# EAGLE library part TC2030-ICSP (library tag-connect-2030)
TAG-CONNECT ICSP Connector Manufacturer: Tag-Connect Cable for easy In-Circuit Serial Programming. Designed for Microchip ICD2, suitable for many others. Two variants - one "with legs" (for hands-free fit on PCB) and another "without legs" for quick programming. PADDescription 1MCLR/Vpp 2Vdd 3GND 4PGD (ISPDAT) 5PGC (ISPCLK) 6nc (used for LVP) ©2009 ROFA.cz - modified and updated by Robert Darlington &#8249;rdarlington@gmail.com&#8250;
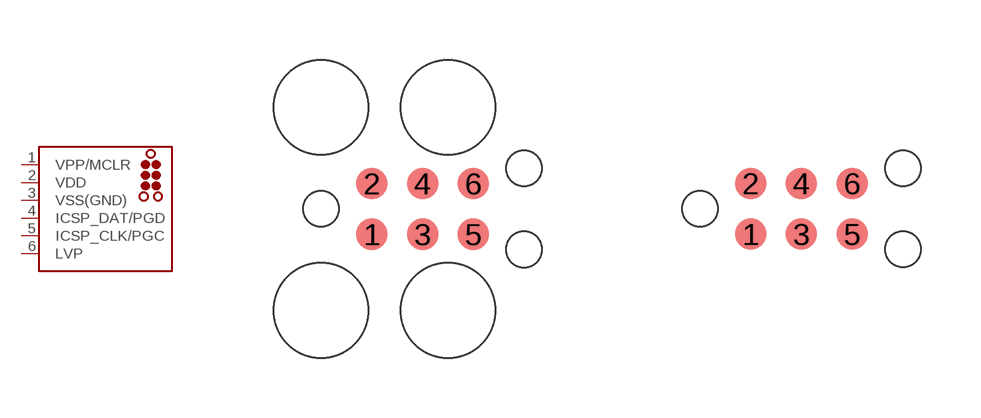
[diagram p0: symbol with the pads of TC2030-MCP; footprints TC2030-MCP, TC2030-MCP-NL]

Designator prefix J

## TC2030-ICSP-MCP  [TC2030-MCP]
1  VPP/MCLR  pas
2  VDD  pwr
3  VSS(GND)  pwr
4  ICSP_DAT/PGD
5  ICSP_CLK/PGC  out
6  LVP

## TC2030-ICSP-MCP-NL  [TC2030-MCP-NL]
Pads as for TC2030-MCP

## TC2030-ICSP  [TC2030-MCP-NL-CP]
Pads as for TC2030-MCP

## Footprint TC2030-MCP (pad centres in mm)
TAG-CONNECT ICSP Connector - Legged version Manufacturer: Tag-Connect Cable for easy In-Circuit Serial Programming. Designed for Microchip ICD2, suitable for many others. NOTE: Eagle's default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
smd 0.787 x 0.787: 1 1.27,-0.635; 2 1.27,0.635; 3 2.54,-0.635; 4 2.54,0.635; 5 3.81,-0.635; 6 3.81,0.635
hole 0.889 at 0,0
hole 0.889 at 5.08,-1.016
hole 0.889 at 5.08,1.016
hole 2.375 at 0,2.54
hole 2.375 at 0,-2.54
hole 2.375 at 3.175,-2.54
hole 2.375 at 3.175,2.54

## Footprint TC2030-MCP-NL (pad centres in mm)
TAG-CONNECT ICSP Connector Manufacturer: Tag-Connect Cable for easy In-Circuit Serial Programming. Designed for Microchip ICD2, suitable for many others. PADDescription 1MCLR/Vpp 2Vdd 3GND 4PGD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
smd 0.787 x 0.787: 1 1.27,-0.635; 2 1.27,0.635; 3 2.54,-0.635; 4 2.54,0.635; 5 3.81,-0.635; 6 3.81,0.635
hole 0.889 at 0,0
hole 0.889 at 5.08,-1.016
hole 0.889 at 5.08,1.016

## Footprint TC2030-MCP-NL-CP (pad centres in mm)
TAG-CONNECT ICSP Connector- with optional copper pads for steel alignment pins Manufacturer: Tag-Connect Cable for easy In-Circuit Serial Programming. Designed for Microchip ICD2, suitable for many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
smd 0.787 x 0.787: 1 1.27,-0.635; 2 1.27,0.635; 3 2.54,-0.635; 4 2.54,0.635; 5 3.81,-0.635; 6 3.81,0.635
hole 1.6 at 0,0
hole 1.6 at 5.08,1.016
hole 1.6 at 5.08,-1.016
